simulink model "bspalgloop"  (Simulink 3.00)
settings: Solver=ode45  StartTime=0.0  StopTime=10.0  FixedStep=0.0001  RelTol=1e-3
libraries: simulink3 x1

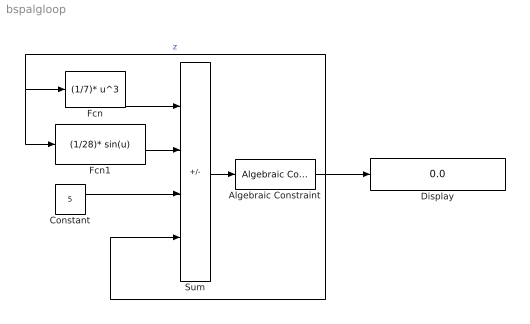
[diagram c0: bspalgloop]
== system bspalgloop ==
  Algebraic Constraint : simulink3/Math/Algebraic Constraint  z0=5
  Constant : Constant  Value=5
  Display : Display
  Fcn : Fcn  Expr=(1/7)* u^3
  Fcn1 : Fcn  Expr=(1/28)* sin(u)
  Sum : Sum  Inputs=+---  SaturateOnIntegerOverflow=on
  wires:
  Fcn/1 -> Sum/1
  Fcn1/1 -> Sum/2
  Constant/1 -> Sum/3
  Sum/1 -> Algebraic Constraint/1
  Algebraic Constraint/1 -> Sum/4, Display/1, Fcn/1, Fcn1/1  "z"
